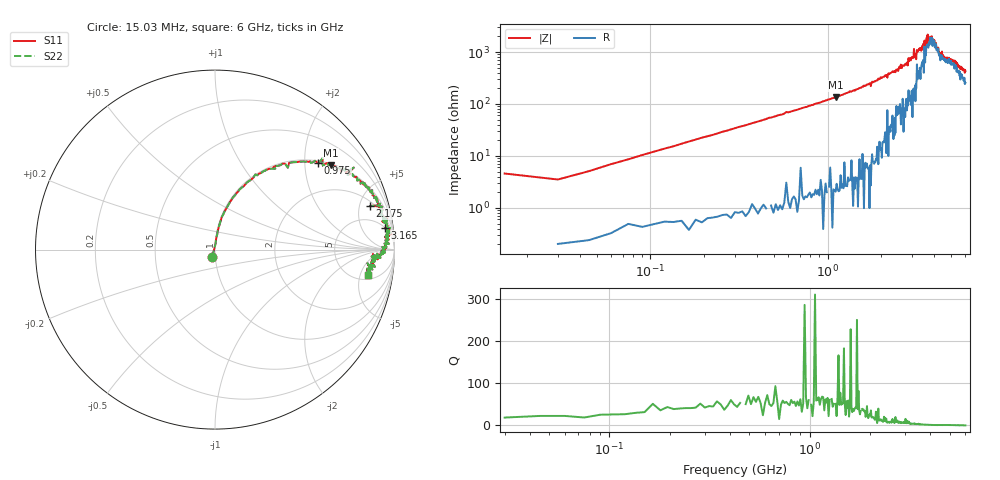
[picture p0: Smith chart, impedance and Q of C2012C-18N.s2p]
!	Network	Analyzer	HP8753E.07.74:	Oct	30	2002	Serial	No.	JP38451487
!	Hewlett-Packard
!	7	Sep	2009	10:46:32
!	Frequency	S11	S21	S12	S22
#	HZ	S	RI	R	50
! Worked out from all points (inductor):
!   400 points, 15.03 MHz to 6 GHz, reference 50 ohm
!   read as one part in series: L = 18.2 nH near 45.03 MHz
!   highest Q = 61.6 at 1.11 GHz (marker M1), where L = 19.4 nH
!   self-resonance near 3.934 GHz
!   S11 on the Smith chart (normalised r, x): 15.03 MHz: 0.97, -0.08; 975 MHz: 1.06, +2.33; 2.175 GHz: 2.52, +6.25; 3.165 GHz: 5, +14; 6 GHz: 6.09, -6.85
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1.502992e7  -0.0159 -0.0431  1.02 0.0431  1.02 0.0431  -0.0159 -0.0431
3.002985e7  0.00348 0.0349  0.997 -0.0349  0.997 -0.0349  0.00348 0.0349
7.502962e7  0.0122 0.0844  0.988 -0.0844  0.988 -0.0844  0.0122 0.0844
1.500292e8  0.0336 0.165  0.966 -0.165  0.966 -0.165  0.0336 0.165
3.150284e8  0.12 0.314  0.88 -0.314  0.88 -0.314  0.12 0.314
9.750251e8  0.574 0.482  0.426 -0.482  0.426 -0.482  0.574 0.482
1.020025e9  0.598 0.48  0.402 -0.48  0.402 -0.48  0.598 0.48
1.110024e9  0.645 0.471  0.355 -0.471  0.355 -0.471  0.645 0.471
2.01002e9  0.898 0.281  0.102 -0.281  0.102 -0.281  0.898 0.281
2.175019e9  0.863 0.243  0.137 -0.243  0.137 -0.243  0.863 0.243
3.015015e9  0.976 0.121  0.0237 -0.121  0.0237 -0.121  0.976 0.121
3.075015e9  0.984 0.0847  0.0162 -0.0847  0.0162 -0.0847  0.984 0.0847
3.165014e9  0.948 0.121  0.0515 -0.121  0.0515 -0.121  0.948 0.121
3.195014e9  0.949 0.0703  0.0512 -0.0703  0.0512 -0.0703  0.949 0.0703
3.495013e9  0.964 0.0772  0.0363 -0.0772  0.0363 -0.0772  0.964 0.0772
3.525012e9  0.954 0.0349  0.0458 -0.0349  0.0458 -0.0349  0.954 0.0349
3.675012e9  0.97 0.0333  0.0297 -0.0333  0.0297 -0.0333  0.97 0.0333
3.705011e9  0.944 0.0337  0.0558 -0.0337  0.0558 -0.0337  0.944 0.0337
4.00501e9  0.947 -0.0164  0.053 0.0164  0.053 0.0164  0.947 -0.0164
4.335008e9  0.905 -0.0547  0.0946 0.0547  0.0946 0.0547  0.905 -0.0547
5.010005e9  0.883 -0.0521  0.117 0.0521  0.117 0.0521  0.883 -0.0521
6e9  0.854 -0.141  0.146 0.141  0.146 0.141  0.854 -0.141
